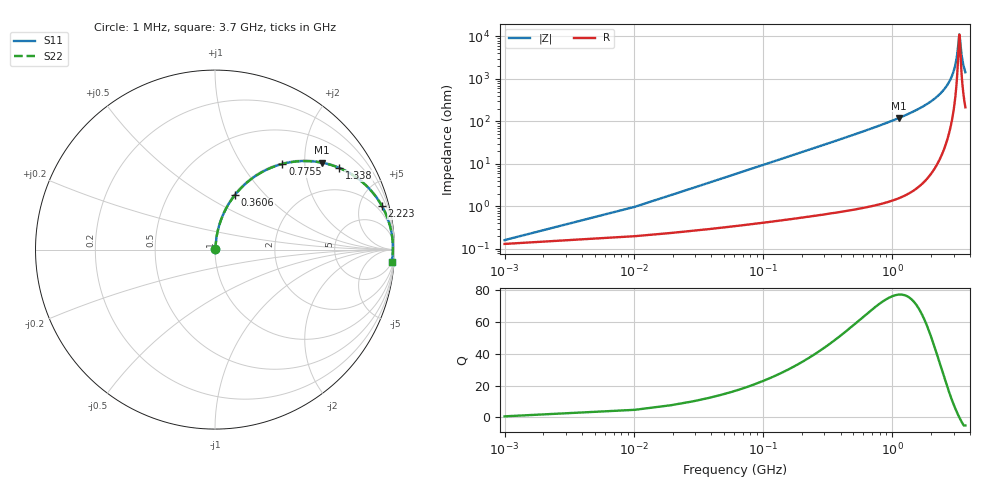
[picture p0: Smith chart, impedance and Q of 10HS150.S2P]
! Coilcraft 1008HS-150 Chip Inductor
! 02 July 2002
# MHZ S MA R 50
!Freq  MagS11  AngS11  MagS21  AngS21  MagS12  AngS12  MagS22  AngS22
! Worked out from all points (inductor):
!   403 points, 1 MHz to 3.7 GHz, reference 50 ohm
!   read as one part in series: L = 15 nH near 19.44 MHz
!   highest Q = 77.2 at 1.135 GHz (marker M1), where L = 17 nH
!   self-resonance near 3.32 GHz
!   S11 on the Smith chart (normalised r, x): 1 MHz: 1.00, +0.00; 360.6 MHz: 1.01, +0.69; 775.5 MHz: 1.02, +1.55; 1.338 GHz: 1.04, +3.01; 2.223 GHz: 1.19, +7.58; 3.7 GHz: 5, -28
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1  0.001613 35.6  0.9987 -0.1  0.9987 -0.1  0.001613 35.6
28.66  0.02706 82.8  0.997 -1.5  0.997 -1.5  0.02706 82.8
37.88  0.0357 83.3  0.9965 -2.0  0.9965 -2.0  0.0357 83.3
56.32  0.05295 83.4  0.9953 -3.0  0.9953 -3.0  0.05295 83.4
83.98  0.07874 82.7  0.9931 -4.5  0.9931 -4.5  0.07874 82.7
185.4  0.1718 78.4  0.98 -9.9  0.98 -9.9  0.1718 78.4
360.58  0.3232 70.0  0.9397 -18.9  0.9397 -18.9  0.3232 70.0
618.74  0.5136 58.2  0.8501 -30.9  0.8501 -30.9  0.5136 58.2
775.48  0.6075 51.8  0.7858 -37.4  0.7858 -37.4  0.6075 51.8
1135.06  0.7663 39.2  0.6327 -50.0  0.6327 -50.0  0.7663 39.2
1236.48  0.7992 36.2  0.5908 -53.0  0.5908 -53.0  0.7992 36.2
1337.9  0.8279 33.4  0.5501 -55.9  0.5501 -55.9  0.8279 33.4
1854.22  0.925 21.4  0.3645 -67.6  0.3645 -67.6  0.925 21.4
2223.02  0.961 14.7  0.2534 -73.9  0.2534 -73.9  0.961 14.7
2471.96  0.9757 10.8  0.1871 -77.2  0.1871 -77.2  0.9757 10.8
2840.76  0.9876 5.7  0.09953 -80.0  0.09953 -80.0  0.9876 5.7
3089.7  0.9908 2.6  0.04679 -77.3  0.04679 -77.3  0.9908 2.6
3191.12  0.9912 1.5  0.02699 -70.3  0.02699 -70.3  0.9912 1.5
3320.2  0.9911 0.0  0.0089 -3.4  0.0089 -3.4  0.9911 0.0
3347.86  0.991 -0.3  0.01014 27.4  0.01014 27.4  0.991 -0.3
3495.38  0.99 -1.8  0.03335 71.6  0.03335 71.6  0.99 -1.8
3700  0.9874 -3.9  0.06862 77.5  0.06862 77.5  0.9874 -3.9
